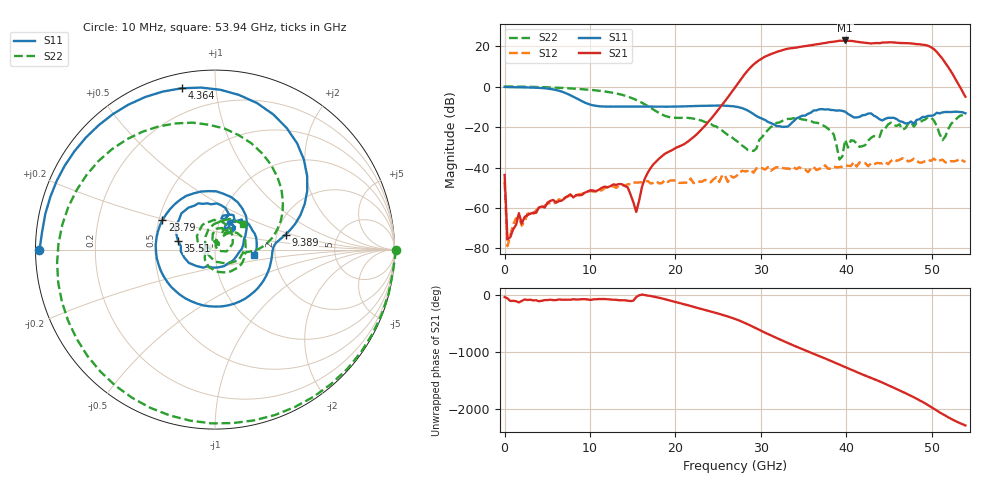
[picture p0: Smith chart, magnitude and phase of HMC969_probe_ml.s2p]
! Hittite Microwave Corporation
! 2 Elizabeth Drive
! Chelmsford, MA 01824
! http://www.hittite.com
! Tel: 978-250-3343
! Fax: 978-250-3373
! Device:  HMC969
! Description: GaAs pHEMT MMIC 1 Watt Power Amplifier
! Frequency:  40.0 - 43.5 GHz
! Package:  DIE
! Ports:  2 RF, 3 DC
!  Pin 1 = RF Input
!  Pin 2 = Vgg
!  Pin 3 = Vdd1
!  Pin 4 = RF Output
!  Pin 5 = Vdd2
!  Pin 6 = Vgg (Alternate)
! Voltages:  Vdd1 = Vdd2 = +6.00 Volts, Idd1 + Idd2 = +894.5 mA
!  Vgg =  -0.77 Volts, Igg =  -6.2 uA
! Data:  The device was measured using G-S-G Probes on a microstrip
!  alumina launch.  The launch is 0.25 inches long. 3 mil Ribbon bonds
!  of approximately 15 mils in length connected the launcher to the die.
!  NO DE_EMBEDDING WAS DONE.
!  Data was collected using an calibrated network analyzer.
!  The reference plane is the microstrip launcher.
! Misc:  Validation Unit  1, +25 C
! Date Measured:  ~2010-10-30
! Date:  2011-11-16 MJV
! Note:
!  Hittite supplies this data as a sample of measured data at the microstrip
!  launch.  Your particular data for this product may vary.
!  Data was taken at 25 degrees C.
!  Hittite reserves the right to change this data at anytime.
# GHZ S DB R 50.0
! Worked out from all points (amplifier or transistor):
!   162 points, 10 MHz to 53.94 GHz, reference 50 ohm
!   highest |S21| = 22.8 dB at 39.87 GHz (marker M1)
!   |S21| within 3 dB of that: 34.88 GHz to 49.75 GHz (14.87 GHz wide, 35.1 % of centre)
!   unconditionally stable (mu >= 1): 309.6 MHz to end of sweep
!   at 9.054 GHz: K = 22296.68, MAG = -46.8 dB, |S12| = -53.0 dB
!   at 27.14 GHz: K = 68.73, MAG = 1.0 dB, |S12| = -44.2 dB
!   at 53.94 GHz: K = 59.32, MAG = -4.6 dB, |S12| = -37.3 dB
!   S11 on the Smith chart (normalised r, x): 10 MHz: 0.01, -0.00; 4.364 GHz: 0.07, +0.81; 9.389 GHz: 2.23, +0.45; 23.79 GHz: 0.52, +0.19; 35.51 GHz: 0.66, +0.07; 53.94 GHz: 1.55, -0.09
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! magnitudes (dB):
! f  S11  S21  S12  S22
! 10 MHz  -0.2  -43.7  -47.1  0.1
! 344.9 MHz  -0.3  -75.5  -78.9  0.0
! 1.35 GHz  -0.3  -68.3  -65.1  0.0
! 4.364 GHz  -0.7  -59.3  -59.8  -0.3
! 9.054 GHz  -7.2  -53.6  -53.0  -1.3
! 9.389 GHz  -7.9  -52.4  -52.5  -1.4
! 13.74 GHz  -9.9  -48.3  -48.6  -4.1
! 15.42 GHz  -9.9  -62.0  -47.5  -6.6
! 18.1 GHz  -10.0  -35.6  -47.9  -13.1
! 23.79 GHz  -9.5  -17.8  -46.7  -18.0
! 27.14 GHz  -10.1  0.5  -44.2  -26.8
! 29.15 GHz  -13.6  10.9  -42.6  -31.8
! 32.5 GHz  -19.9  17.9  -40.2  -17.0
! 35.51 GHz  -13.5  20.2  -42.3  -16.7
! 36.18 GHz  -11.8  20.6  -39.7  -17.7
! 38.53 GHz  -11.7  22.1  -39.6  -23.7
! 39.2 GHz  -11.8  22.6  -39.8  -36.1
! 39.87 GHz  -12.4  22.8  -38.9  -26.3
! 45.23 GHz  -15.4  21.9  -36.7  -17.9
! 50.25 GHz  -14.1  18.5  -35.6  -16.8
! 51.26 GHz  -12.8  13.7  -36.1  -26.5
! 53.94 GHz  -13.3  -5.0  -37.3  -13.6
